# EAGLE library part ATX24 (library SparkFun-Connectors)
ATX24 Pin Power Supply Connector - Right Angle PTH Mount This is a good connector for connecting a computer power supply to a PCB. It's massive, but provides many amps of power at 5V and 12V. SparkFun Products: SparkFun Benchtop Power Board Kit SparkFun Power Driver Shield Kit
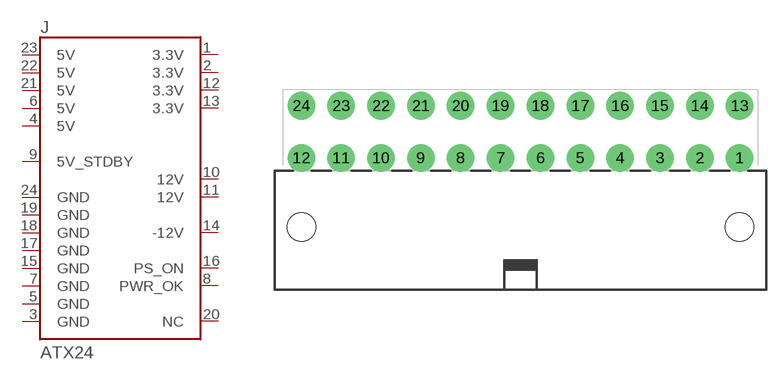
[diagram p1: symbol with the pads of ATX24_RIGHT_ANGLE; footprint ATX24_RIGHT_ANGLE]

Designator prefix J

## ATX24RH (PROD_ID: CONN-09674; SF_ID: PRT-09498)  [ATX24_RIGHT_ANGLE]
1  3.3V
2  3.3V
3  GND
4  5V
5  GND
6  5V
7  GND
8  PWR_OK
9  5V_STDBY
10  12V
11  12V
12  3.3V
13  3.3V
14  -12V
15  GND
16  PS_ON
17  GND
18  GND
19  GND
20  NC
21  5V
22  5V
23  5V
24  GND

## Footprint ATX24_RIGHT_ANGLE (pad centres in mm)
Molex Mini-Fit Jr. - 24 pin, Right Angle Specifications: Pin count:24 Datasheet referenced for footprint Example device(s): ATX24
drill 1.8 pad 2.9: 1 23.1,4.76; 2 18.9,4.76; 3 14.7,4.76; 4 10.5,4.76; 5 6.3,4.76; 6 2.1,4.76; 7 -2.1,4.76; 8 -6.3,4.76; 9 -10.5,4.76; 10 -14.7,4.76; 11 -18.9,4.76; 12 -23.1,4.76; 13 23.1,10.26; 14 18.9,10.26; 15 14.7,10.26; 16 10.5,10.26; 17 6.3,10.26; 18 2.1,10.26; 19 -2.1,10.26; 20 -6.3,10.26; 21 -10.5,10.26; 22 -14.7,10.26; 23 -18.9,10.26; 24 -23.1,10.26
hole 3 at -23.1,-2.54
hole 3 at 23.1,-2.54

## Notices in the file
Licensing: Creative Commons ShareAlike 4.0 International - https://creativecommons.org/licenses/by-sa/4.0
